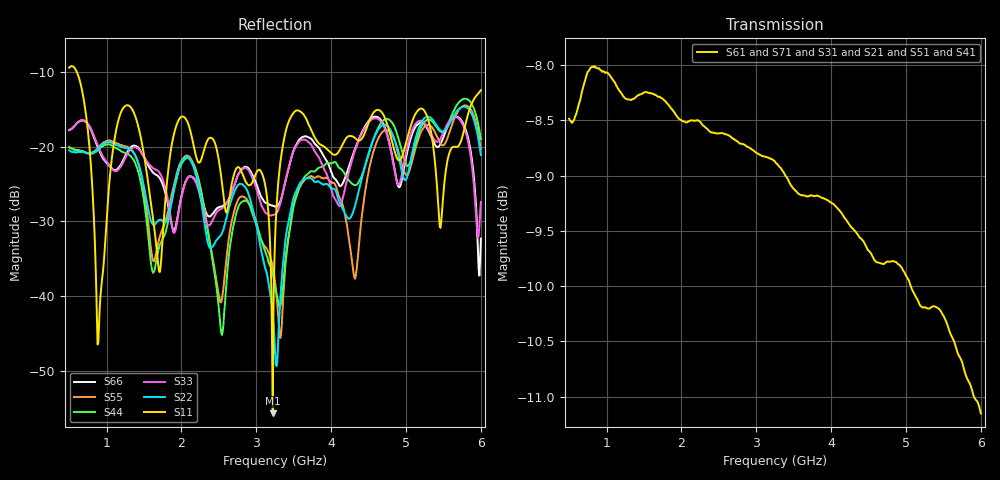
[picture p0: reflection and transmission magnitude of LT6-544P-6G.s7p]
! MTS Systemtechnik GmbH
! S-Parameters
! Model: LT6-544P-6G
! Rohde & Schwarz ZVB8 2Ports - Version 3.20 - 1145.1010k08 SN: 100119
! Converted & adapted with Octave
!		|  MTS  |
!		|  |--o OUT 6 (Port 7)
!		|  |--o OUT 5 (Port 6)
!		|  |--o OUT 4 (Port 5)
! C (Port 1) o--|  LT6-544P-6G  |
!		|  |--o OUT 3 (Port 4)
!		|  |--o OUT 2 (Port 3)
!  |  |--o OUT 1 (Port 2)
! S7P File: Measurements:
! <S11,S12,S13,S14,S15,S16,S17>,
! <S21,S22,S23,S24,S25,S26,S27>,
! <S31,S32,S33,S34,S35,S36,S37>,
! <S41,S42,S43,S44,S45,S46,S47>,
! <S51,S52,S53,S54,S55,S56,S57>,
! <S61,S62,S63,S64,S65,S66,S67>,
! <S71,S72,S73,S74,S75,S76,S77>:
# HZ  S  DB  R  50.00
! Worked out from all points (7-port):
!   551 points, 500 MHz to 6 GHz, reference 50 ohm
!   strongest paths, dB at 500 MHz, 1.87 GHz, 3.25 GHz, 4.63 GHz, 6 GHz:
!     S61: -8.5, -8.4, -8.9, -9.8, -11.2
!     S71: -8.5, -8.5, -8.9, -9.9, -11.2
!     S31: -8.5, -8.4, -8.9, -9.8, -11.3
!     S21: -8.5, -8.5, -9.0, -10.0, -11.4
!     S51: -8.5, -8.5, -9.0, -9.9, -11.5
!     S41: -8.5, -8.5, -9.0, -9.9, -11.4
!   lowest |S11| = -55.7 dB at 3.22 GHz (marker M1), VSWR 1.00, Z = 50.1 + j0.143 ohm
!   |S11| at or under -10 dB: 603 MHz to end of sweep
